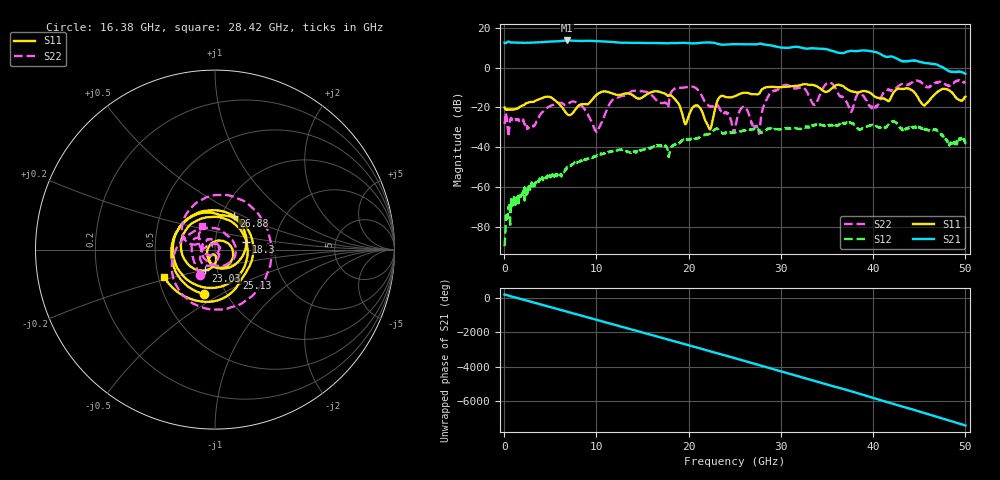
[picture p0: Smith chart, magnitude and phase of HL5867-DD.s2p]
! 3/25/2021 10:01:04 AM
! H:\PRODUCTION_DATA\TEMP_S2P.S2P
! CHANNEL.1
! TR.MEASUREMENT
! CORRECTED.DATA
# GHZ S RI R 50.0
! FREQ.GHZ  S11RE  S11IM  S21RE  S21IM  S12RE  S12IM  S22RE  S22IM
!; PortSelection: Port_12
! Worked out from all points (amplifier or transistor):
!   1429 points, 35 MHz to 50.02 GHz, reference 50 ohm
!   highest |S21| = 13.7 dB at 6.825 GHz (marker M1)
!   |S21| within 3 dB of that: start of sweep to 29.43 GHz
!   unconditionally stable (mu >= 1): start of sweep to end of sweep
!   at 8.365 GHz: K = 23.10, MAG = 13.5 dB, |S12| = -46.9 dB
!   at 25.02 GHz: K = 5.12, MAG = 12.0 dB, |S12| = -32.3 dB
!   at 50.02 GHz: K = 47.34, MAG = -2.0 dB, |S12| = -38.6 dB
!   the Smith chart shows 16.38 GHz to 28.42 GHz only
!   S11 on the Smith chart (normalised r, x): 16.38 GHz: 0.79, -0.42; 18.3 GHz: 1.42, +0.13; 23.03 GHz: 0.88, -0.21; 25.13 GHz: 1.21, -0.39; 26.88 GHz: 1.14, +0.45; 28.42 GHz: 0.54, -0.18
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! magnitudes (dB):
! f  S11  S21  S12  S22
! 35 MHz  -20.0  12.6  -89.7  -28.3
! 1.26 GHz  -20.8  12.6  -64.8  -25.9
! 6.825 GHz  -23.3  13.7  -49.8  -18.7
! 8.365 GHz  -18.4  13.4  -46.9  -19.0
! 10.01 GHz  -13.6  13.4  -44.2  -32.3
! 11.97 GHz  -13.4  12.8  -41.4  -15.4
! 16.38 GHz  -11.9  12.4  -39.3  -15.7
! 16.7 GHz  -12.0  12.4  -38.8  -17.0
! 18.3 GHz  -14.9  12.4  -38.8  -11.1
! 22.23 GHz  -30.5  12.6  -33.2  -19.2
! 23.03 GHz  -17.9  12.2  -30.8  -18.7
! 25.02 GHz  -14.3  11.8  -32.3  -31.0
! 25.13 GHz  -14.1  11.9  -32.5  -28.3
! 25.97 GHz  -12.6  11.8  -31.8  -19.8
! 26.88 GHz  -13.3  11.7  -30.9  -27.7
! 28.42 GHz  -9.9  11.5  -31.1  -16.3
! 30.59 GHz  -9.6  10.0  -30.2  -8.8
! 33.39 GHz  -8.6  9.7  -29.0  -17.6
! 35.21 GHz  -11.7  9.0  -29.0  -7.5
! 37.59 GHz  -11.8  8.4  -27.6  -22.1
! 41.69 GHz  -16.8  5.5  -28.4  -11.3
! 50.02 GHz  -14.6  -3.1  -38.6  -7.3
